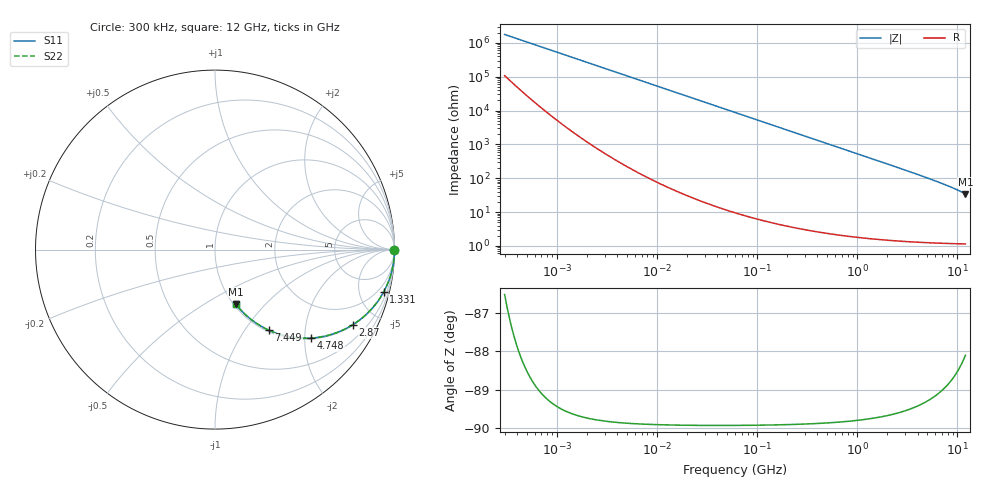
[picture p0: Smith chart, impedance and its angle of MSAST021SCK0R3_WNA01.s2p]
! MSAST021SCK0R3_WNA01  S-PARAMETER MODEL  ( General Type )
! Model Generated by TAIYO YUDEN Corporation (http://www.ty-top.com)
! Version 2.0
! TAIYO YUDEN Control No. 181101
! Copyright(c) 2015 TAIYO YUDEN CO.,LTD. All Rights Reserved.
! Product Description (link to TY-COMPAS)
! https://ds.yuden.co.jp/TYCOMPAS/or/detail?pn=MSAST021SCK0R3BWNA01&u=M
! Products Name : Multilayer Ceramic Capacitors
! Characteristics :
!  Capacitance : 0.3 pF , Rated Voltage : 25V , TCC : CK / C0K
!  Case Size : 0.25 x 0.125 / 0.0098 x 0.0049 [mm/inch] , Thickness : 0.125 / 0.0049 [mm/inch]
!  (Conditions: Temperature = 25 degC , DC Bias Current/Voltage = 0A / 0V)
! External Node Assignments :
!  1  o---| |---o  2
! GND o---------o GND
! Frequency Range : 0.3MHz  -  12000MHz  [ 401 STEP ]
# MHz S RI R 50
! Freq[MHz].  S11 Real  S11 Imag  S21 Real  S21 Imag  S12 Real  S12 Imag  S22 Real  S22 Imag
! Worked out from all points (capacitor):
!   401 points, 300 kHz to 12 GHz, reference 50 ohm
!   read as one part in series: C = 301 fF near 316.3 kHz
!   lowest |Z| = 34.6 ohm at 12 GHz (marker M1)
!   S11 on the Smith chart (normalised r, x): 300 kHz: open; 1.331 GHz: 1.03, -7.93; 2.87 GHz: 1.03, -3.64; 4.748 GHz: 1.03, -2.15; 7.449 GHz: 1.02, -1.30; 12 GHz: 1.02, -0.69
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0.3  1 -5.64e-05  3.45e-06 5.64e-05  3.45e-06 5.64e-05  1 -5.64e-05
0.496271  1 -9.37e-05  2.46e-06 9.37e-05  2.46e-06 9.37e-05  1 -9.37e-05
0.537322  1 -0.000101  2.36e-06 0.000101  2.36e-06 0.000101  1 -0.000101
1.769972  1 -0.000334  1.79e-06 0.000334  1.79e-06 0.000334  1 -0.000334
10.44266  1 -0.00197  6.66e-06 0.00197  6.66e-06 0.00197  1 -0.00197
60  0.9999 -0.0113  0.000141 0.0113  0.000141 0.0113  0.9999 -0.0113
164.1901  0.999 -0.031  0.001 0.031  0.001 0.031  0.999 -0.031
353.9943  0.9954 -0.0666  0.00457 0.0666  0.00457 0.0666  0.9954 -0.0666
512.9422  0.9905 -0.096  0.00952 0.096  0.00952 0.096  0.9905 -0.096
723.8279  0.9813 -0.1342  0.0187 0.1342  0.0187 0.1342  0.9813 -0.1342
994.7115  0.9652 -0.1815  0.0348 0.1815  0.0348 0.1815  0.9652 -0.1815
1331.232  0.9394 -0.2366  0.0606 0.2366  0.0606 0.2366  0.9394 -0.2366
1689.663  0.9057 -0.2898  0.0943 0.2898  0.0943 0.2898  0.9057 -0.2898
2088.533  0.8624 -0.3416  0.1376 0.3416  0.1376 0.3416  0.8624 -0.3416
2870.14  0.7668 -0.4191  0.2332 0.4191  0.2332 0.4191  0.7668 -0.4191
3740.715  0.6562 -0.4703  0.3438 0.4703  0.3438 0.4703  0.6562 -0.4703
4747.894  0.5368 -0.4929  0.4632 0.4929  0.4632 0.4929  0.5368 -0.4929
5868.704  0.4236 -0.4871  0.5764 0.4871  0.5764 0.4871  0.4236 -0.4871
7448.838  0.3013 -0.4498  0.6987 0.4498  0.6987 0.4498  0.3013 -0.4498
9708.23  0.1857 -0.3767  0.8143 0.3767  0.8143 0.3767  0.1857 -0.3767
11380.75  0.1305 -0.3219  0.8695 0.3219  0.8695 0.3219  0.1305 -0.3219
12000  0.1146 -0.3024  0.8854 0.3024  0.8854 0.3024  0.1146 -0.3024
